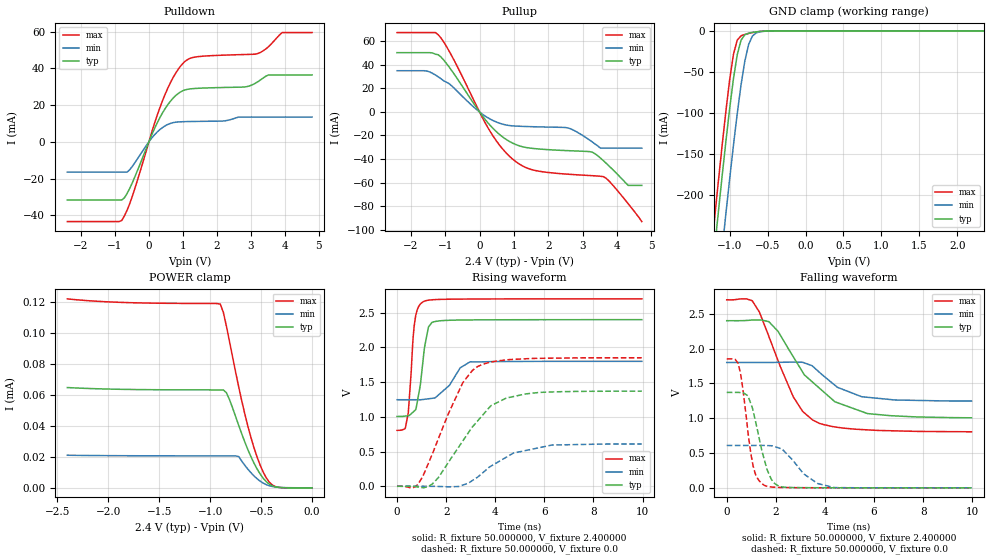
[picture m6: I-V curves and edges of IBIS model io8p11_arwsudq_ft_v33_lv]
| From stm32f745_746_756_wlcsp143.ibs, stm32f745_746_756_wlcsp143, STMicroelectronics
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|   Model io8p11_arwsudq_ft_v33_lv
[Model]  io8p11_arwsudq_ft_v33_lv
Model_type I/O
Polarity   Non-Inverting
Enable   Active-Low
Vinl =   0.720000V
Vinh =   1.680000V
Vmeas =  1.200000V
Cref =   30.000000pF
Rref =   100.000000M
Vref =   0.0V
C_comp   2.828400pF   2.777000pF   2.910300pF
[Temperature Range]   25.000000   0.125000k   -40.000000
[Pullup Reference]   2.400000V   1.800000V   2.700000V
[Pulldown Reference]   0.0V   0.0V   0.0V
[POWER Clamp Reference]   2.400000V   1.800000V   2.700000V
[GND Clamp Reference]   0.0V   0.0V   0.0V
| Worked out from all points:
|   slope of the pulldown table from 0 to 0.36 V, typ, clamps not added: 25 ohm
|   slope of the pullup table from 0 to 0.36 V, typ, clamps not added: 27.7 ohm
|   GND clamp passes 1 mA (typ) near -0.62 V on its own axis
|   rising waveform, R_fixture 50.000000, V_fixture 2.400000: 20-80 % time 324ps typ, 721ps min, 219ps max; typ from 1.01 V to 2.4 V
|   rising waveform, R_fixture 50.000000, V_fixture 0.0: 20-80 % time 1.7ns typ, 1.63ns min, 1.34ns max; typ from 0 V to 1.37 V
|   falling waveform, R_fixture 50.000000, V_fixture 2.400000: 20-80 % time 1.95ns typ, 1.46ns min, 1.38ns max; typ from 2.4 V to 1.01 V
|   falling waveform, R_fixture 50.000000, V_fixture 0.0: 20-80 % time 553ps typ, 1.01ns min, 414ps max; typ from 1.37 V to 0 V
[Pulldown]
|Voltage   I(typ)   I(min)   I(max)
-2.4V     -31.66mA   -16.51mA   -43.43mA
-800mV    -31.66mA   -16.51mA   -42.86mA
-480mV    -21.98mA   -13.17mA   -29.21mA
80mV      3.63mA     1.966mA    5.014mA
480mV     18.16mA    8.738mA    26.02mA
800mV     25.38mA    10.72mA    37.77mA
1.12V     28.53mA    11.02mA    44.6mA
2.8V      29.84mA    13.48mA    47.53mA
3.2V      32.65mA    13.48mA    48.04mA
3.52V     36.42mA    13.48mA    51.83mA
3.92V     36.42mA    13.48mA    59.49mA
4.8V      36.42mA    13.48mA    59.49mA
[Pullup]
|Voltage   I(typ)   I(min)   I(max)
-2.4V     50.45mA    35.09mA    67.53mA
-1.52V    50.45mA    34.74mA    67.53mA
-1.2V     48.64mA    29.86mA    65.66mA
-800mV    34.82mA    21.94mA    47.28mA
320mV     -11.75mA   -6.207mA   -17.08mA
1.04V     -27.54mA   -11.97mA   -41.91mA
1.6V      -31.14mA   -12.58mA   -49.63mA
2.56V     -32.88mA   -13.49mA   -52.9mA
3.28V     -34.2mA    -25.51mA   -54.18mA
3.6V      -41.34mA   -30.76mA   -55mA
4.32V     -62.43mA   -30.76mA   -77.88mA
4.72V     -62.43mA   -30.76mA   -93.2mA
[GND_clamp]
|Voltage   I(typ)   I(min)   I(max)
-2.4V     -1.428A    -1.51A     -1.4A
-1.2V     -266.4mA   -356.3mA   -229.4mA
-1.15V    -221.3mA   -311mA     -184.1mA
-1.1V     -177.3mA   -266.4mA   -140mA
-1.05V    -134.8mA   -222.7mA   -97.97mA
-950mV    -58.22mA   -139.2mA   -28.55mA
-900mV    -29.03mA   -100.6mA   -11.27mA
-850mV    -11.41mA   -65.77mA   -6.067mA
-750mV    -2.852mA   -16.63mA   -3.179mA
-700mV    -1.914mA   -6.318mA   -2.181mA
-600mV    -750uA     -1.167mA   -738.3uA
2.35V     0A         0A         0A
[POWER_clamp]
|Voltage   I(typ)   I(min)   I(max)
-2.4V     64.71uA    21.03uA    121.9uA
-1.86V    63.55uA    20.74uA    119.6uA
-900mV    63.18uA    20.63uA    118.5uA
-870mV    63.14uA    20.63uA    113.2uA
-840mV    61.36uA    20.62uA    104.3uA
-720mV    40.37uA    20.18uA    65.28uA
-630mV    24.69uA    12.08uA    39.85uA
-540mV    12.26uA    5.907uA    20uA
-480mV    6.236uA    3.061uA    10.23uA
-420mV    2.4uA      1.365uA    3.726uA
-360mV    667.9nA    564nA      839.6nA
0V        0A         0A         0A
[Ramp]
| variable   typ   min   max
dV/dt_r  0.82182/1.69966n   0.36957/1.70435n   1.11138/1.33767n
dV/dt_f  0.83586/1.95403n   0.33210/1.46344n   1.13598/1.37986n
R_load = 50.000000
[Rising Waveform]
R_fixture= 50.000000
V_fixture= 2.400000
V_fixture_min= 1.800000
V_fixture_max= 2.700000
|time   V(typ)   V(min)   V(max)
0s        1.006V     1.247V     804.9mV
340.3ps   1.011V     1.247V     841.7mV
460.5ps   1.016V     1.247V     1.065V
660.7ps   1.071V     1.247V     2.164V
740.7ps   1.096V     1.247V     2.413V
1.081ns   1.883V     1.251V     2.661V
1.281ns   2.294V     1.26V      2.681V
1.642ns   2.379V     1.301V     2.691V
2.983ns   2.396V     1.793V     2.697V
9.97ns    2.4V       1.8V       2.7V
[Rising Waveform]
R_fixture= 50.000000
V_fixture= 0.0
V_fixture_min= 0.0
V_fixture_max= 0.0
|time   V(typ)   V(min)   V(max)
0s        77uV       34.87uV    227.1uV
620.6ps   -2.464mV   18.8uV     -22.77mV
860.9ps   -11.17mV   63.75uV    32.54mV
1.441ns   33.8mV     -758.8uV   467.8mV
2.663ns   644.2mV    15.07mV    1.48V
3.283ns   941.4mV    131.6mV    1.726V
3.824ns   1.161V     289.4mV    1.789V
5.265ns   1.331V     516.8mV    1.837V
6.306ns   1.359V     594mV      1.845V
9.97ns    1.37V      609.1mV    1.851V
[Falling Waveform]
R_fixture= 50.000000
V_fixture= 2.400000
V_fixture_min= 1.800000
V_fixture_max= 2.700000
|time   V(typ)   V(min)   V(max)
0s        2.4V       1.8V       2.7V
1.041ns   2.409V     1.8V       2.685V
1.341ns   2.41V      1.8V       2.514V
1.722ns   2.384V     1.8V       2.169V
2.703ns   1.886V     1.805V     1.313V
3.163ns   1.622V     1.794V     1.076V
3.504ns   1.516V     1.745V     973.2mV
4.404ns   1.236V     1.474V     874.4mV
5.506ns   1.095V     1.308V     836.8mV
9.97ns    1.006V     1.247V     804.9mV
[Falling Waveform]
R_fixture= 50.000000
V_fixture= 0.0
V_fixture_min= 0.0
V_fixture_max= 0.0
|time   V(typ)   V(min)   V(max)
0s        1.37V      609.1mV    1.851V
460.5ps   1.371V     609mV      1.789V
660.7ps   1.366V     608.9mV    1.41V
860.9ps   1.323V     608.9mV    813mV
1.161ns   971.2mV    608.7mV    204.7mV
1.542ns   391.9mV    608.7mV    34.64mV
2.122ns   26.51mV    572.3mV    6.46mV
3.143ns   2.514mV    198.3mV    1.983mV
4.384ns   1.112mV    3.765mV    946uV
9.97ns    77uV       34.87uV    227.1uV
